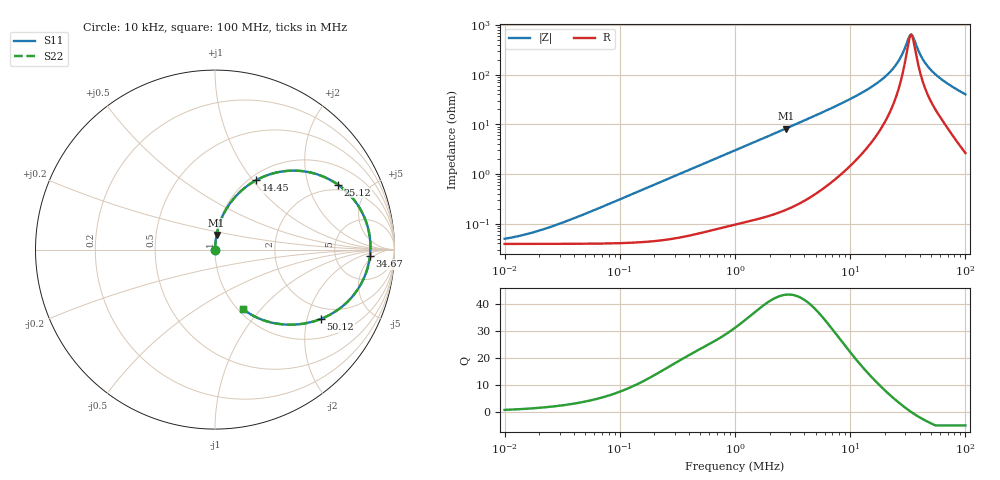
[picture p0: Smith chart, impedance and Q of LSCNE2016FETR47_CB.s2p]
! LSCNE2016FETR47_CB  S-PARAMETER MODEL  ( Standard Model )
! Model Generated by TAIYO YUDEN Corporation (http://www.ty-top.com)
! Version 1.0
! TAIYO YUDEN Control No. 200220
! Copyright(c) 2020 TAIYO YUDEN CO.,LTD. All Rights Reserved.
! Product Description (link to TY-COMPAS)
! https://ds.yuden.co.jp/TYCOMPAS/or/detail?pn=LSCNE2016FETR47MCB&u=M
! Products Name : Inductors
! Characteristics :
!  Inductance : 0.47 [uH] , SRF(min) : - [Hz] , DC Resistance(max) : 45 [mOhm]
!  Rated Current : Saturation  4.0 [A] (dL = 30 [%]), Temp Rise  3.2 [A] (dT = 40 [degC])
!  Case Size : 2.0 x 1.6 / 0.079 x 0.063 [mm/inch] , Thickness : 0.65 / 0.026 [mm/inch]
!  (Conditions: Temperature = 25 [degC] , DC Bias Current = 0 [A])
! External Node Assignments :
!  1  o---GGG---o  2
! GND o---------o GND
! Frequency Range : 10kHz  -  100MHz  [ 402 STEP ]
# MHz S RI R 50
! Freq[MHz].  S11 Real  S11 Imag  S21 Real  S21 Imag  S12 Real  S12 Imag  S22 Real  S22 Imag
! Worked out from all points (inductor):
!   401 points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, 10 kHz to 100 MHz, reference 50 ohm
!   read as one part in series: L = 485 nH near 38.91 kHz
!   highest Q = 43.6 at 2.754 MHz (marker M1), where L = 474 nH
!   self-resonance near 33.85 MHz
!   S11 on the Smith chart (normalised r, x): 10 kHz: 1.00, +0.00; 14.45 MHz: 1.07, +1.04; 25.12 MHz: 1.74, +3.14; 34.67 MHz: 13, -4; 50.12 MHz: 1.58, -2.43; 100 MHz: 1.05, -0.80
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0.01  0.000389 0.000304  0.9996 -0.000304  0.9996 -0.000304  0.000389 0.000304
0.019953  0.00039 0.000607  0.9996 -0.000607  0.9996 -0.000607  0.00039 0.000607
0.046774  0.000394 0.00142  0.9996 -0.00142  0.9996 -0.00142  0.000394 0.00142
0.218776  0.000497 0.00664  0.9995 -0.00664  0.9995 -0.00664  0.000497 0.00664
1  0.00184 0.0298  0.9982 -0.0298  0.9982 -0.0298  0.00184 0.0298
2.754229  0.00851 0.0811  0.9915 -0.0811  0.9915 -0.0811  0.00851 0.0811
4.677351  0.0228 0.1371  0.9772 -0.1371  0.9772 -0.1371  0.0228 0.1371
9.120108  0.0867 0.2617  0.9133 -0.2617  0.9133 -0.2617  0.0867 0.2617
14.4544  0.2292 0.3866  0.7708 -0.3866  0.7708 -0.3866  0.2292 0.3866
17.78279  0.3566 0.4323  0.6434 -0.4323  0.6434 -0.4323  0.3566 0.4323
21.87762  0.5413 0.4273  0.4587 -0.4273  0.4587 -0.4273  0.5413 0.4273
25.11886  0.6849 0.3619  0.3151 -0.3619  0.3151 -0.3619  0.6849 0.3619
28.18383  0.7921 0.2533  0.2079 -0.2533  0.2079 -0.2533  0.7921 0.2533
32.35937  0.8629 0.0669  0.1371 -0.0669  0.1371 -0.0669  0.8629 0.0669
33.88442  0.866 -0.00143  0.134 0.00143  0.134 0.00143  0.866 -0.00143
34.67368  0.8635 -0.0354  0.1365 0.0354  0.1365 0.0354  0.8635 -0.0354
41.68694  0.7607 -0.2671  0.2393 0.2671  0.2393 0.2671  0.7607 -0.2671
45.70882  0.6768 -0.3409  0.3232 0.3409  0.3232 0.3409  0.6768 -0.3409
50.11872  0.5894 -0.3866  0.4106 0.3866  0.4106 0.3866  0.5894 -0.3866
58.88437  0.4489 -0.4174  0.5511 0.4174  0.5511 0.4174  0.4489 -0.4174
70.79458  0.318 -0.4074  0.682 0.4074  0.682 0.4074  0.318 -0.4074
100  0.1548 -0.3303  0.8452 0.3303  0.8452 0.3303  0.1548 -0.3303
